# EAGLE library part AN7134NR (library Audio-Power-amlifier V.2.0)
Dual 7,5W Audio Power Ampliefier
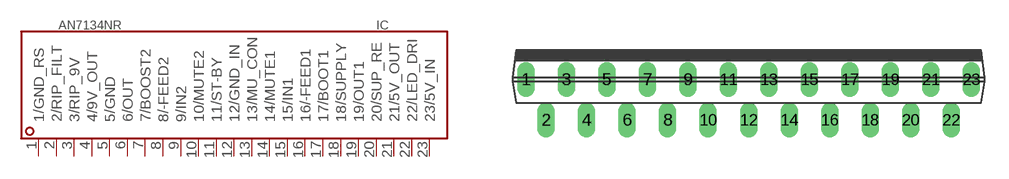
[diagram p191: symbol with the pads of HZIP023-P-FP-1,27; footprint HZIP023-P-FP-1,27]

Designator prefix IC

## AN7134NR  [HZIP023-P-FP-1,27]
1  1/GND_RS  pwr
2  2/RIP_FILT  in
3  3/RIP_9V  in
4  4/9V_OUT  out
5  5/GND  out
6  6/OUT  out
7  7/BOOST2  out
8  8/-FEED2  in
9  9/IN2  in
10  10/MUTE2  out
11  11/ST-BY  in
12  12/GND_IN  pwr
13  13/MU_CON  in
14  14/MUTE1  out
15  15/IN1  in
16  16/-FEED1  in
17  17/BOOT1  in
18  18/SUPPLY  pwr
19  19/OUT1  out
20  20/SUP_RE  pwr
21  21/5V_OUT  out
22  22/LED_DRI  out
23  23/5V_IN  in

## Footprint HZIP023-P-FP-1,27 (pad centres in mm)
23-Lead ZSIL Plastic package with FIN
drill 0.6 long: 1 -13.97,0; 2 -12.7,-2.54; 3 -11.43,0; 4 -10.16,-2.54; 5 -8.89,0; 6 -7.62,-2.54; 7 -6.35,0; 8 -5.08,-2.54; 9 -3.81,0; 10 -2.54,-2.54; 11 -1.27,0; 12 0,-2.54; 13 1.27,0; 14 2.54,-2.54; 15 3.81,0; 16 5.08,-2.54; 17 6.35,0; 18 7.62,-2.54; 19 8.89,0; 20 10.16,-2.54; 21 11.43,0; 22 12.7,-2.54; 23 13.97,0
